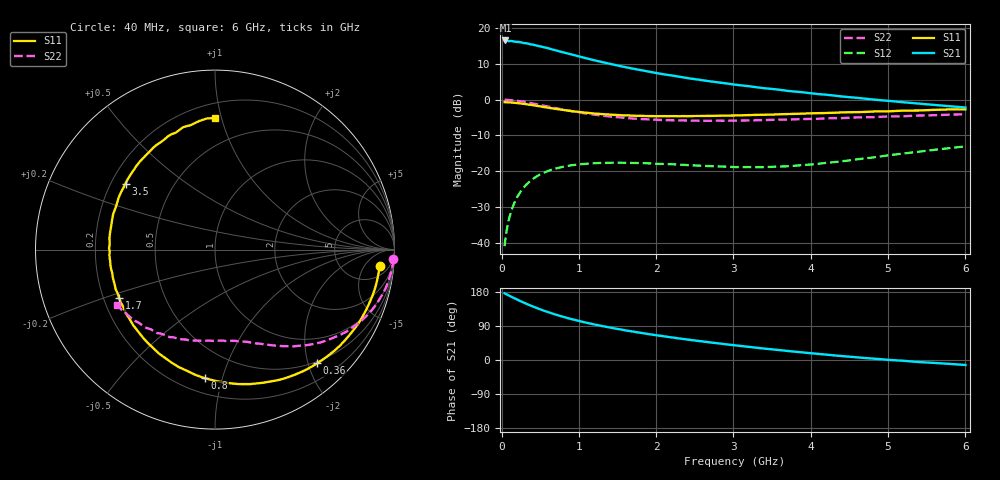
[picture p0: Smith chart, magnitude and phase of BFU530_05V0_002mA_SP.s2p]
! Filename:  P:\Prog\Test\Noise\ATS_data\Testdata_Net\03 Spar\BFU530_APG2013_40_A05_05p0V_002mA_SP_CM01_D.s2p
! Date/Time: Fri 26/Apr/2013 13:03:15
! BFU530_APG2013_40_A05_05p0V_1to25mA_SP_CM01_Bias2_R.s2p
! MDIF S-parameter v. bias file
! BFU530_APG2013_40_A05_05p0V_1to25mA_SP_CM01
! Date/time Wed Apr 24 19:36:53 2013
! VAR V_out= 5.0000
! VAR I_out= 1.9900
! VAR V_in= 0.7986
! VAR I_in= 0.0213
! Device data file deembeded for feedlines and parallel
! Original file: \03 Spar\BFU530_APG2013_40_A05_05p0V_002mA_SP_CM01_R.s2p
! Feed-files: PR047V01_250413_Feed1.s2p, PR047V01_250413_Feed2.s2p
! Parallel-file: PR047V01_250413_Par.s2p
# MHz S MA R 50
!  Freq-MHz  S11-mag  S11-arg  S21-mag  S21-arg  S12-mag  S12-arg  S22-mag  S22-arg
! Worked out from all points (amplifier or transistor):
!   98 points, 40 MHz to 6 GHz, reference 50 ohm
!   highest |S21| = 16.6 dB at 50 MHz (marker M1)
!   |S21| within 3 dB of that: start of sweep to 740.2 MHz
!   unconditionally stable (mu >= 1): 2.879 GHz to 4.826 GHz
!   at 300 MHz: K = 0.11, MSG = 20.0 dB, |S12| = -24.2 dB
!   at 1.6 GHz: K = 0.54, MSG = 13.4 dB, |S12| = -17.6 dB
!   at 6 GHz: K = 0.81, MSG = 5.4 dB, |S12| = -13.0 dB
!   S11 on the Smith chart (normalised r, x): 40 MHz: 10, -12; 360 MHz: 0.47, -2.16; 800 MHz: 0.30, -0.88; 1.7 GHz: 0.26, -0.22; 3.5 GHz: 0.26, +0.31; 6 GHz: 0.30, +0.95
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40  0.9241 -5.6  6.71 176.0  0.008973 86.3  0.9957 -3.0
50  0.9221 -6.9  6.73 174.4  0.01118 85.5  0.9959 -3.8
60  0.9208 -8.1  6.643 173.7  0.01341 84.9  0.9948 -4.7
120  0.9142 -16.6  6.629 167.6  0.02641 79.8  0.9843 -9.2
240  0.887 -32.8  6.374 155.8  0.05061 70.1  0.9517 -18.2
360  0.8517 -48.1  6.017 145.1  0.07123 61.4  0.9054 -26.2
440  0.8265 -57.6  5.761 138.4  0.08274 56.3  0.8706 -30.9
550  0.7886 -70.2  5.403 129.9  0.09555 49.7  0.8212 -36.8
700  0.7446 -85.4  4.905 119.8  0.109 42.3  0.7622 -43.5
800  0.7188 -94.6  4.589 113.8  0.1157 38.2  0.7258 -47.4
900  0.6928 -103.2  4.301 108.2  0.1211 34.5  0.6958 -50.8
1050  0.6642 -114.9  3.905 100.6  0.126 29.6  0.6518 -55.5
1200  0.6411 -125.4  3.562 93.8  0.1293 25.6  0.6183 -59.5
1350  0.6237 -134.6  3.265 87.7  0.131 22.4  0.5908 -63.1
1700  0.5981 -153.3  2.719 75.1  0.1305 17.0  0.5452 -70.5
2050  0.5887 -169.1  2.31 64.0  0.1268 13.9  0.5211 -77.4
2500  0.5918 173.9  1.939 51.5  0.1206 13.1  0.509 -85.8
3100  0.6043 154.3  1.585 36.9  0.1143 17.5  0.5118 -96.8
3500  0.6197 143.6  1.414 28.1  0.1155 22.7  0.5232 -104.2
4100  0.6483 128.0  1.198 16.0  0.1271 30.6  0.5413 -115.5
5200  0.705 104.5  0.921 -2.1  0.1772 35.9  0.5877 -135.9
6000  0.7332 90.2  0.7785 -13.1  0.2228 32.5  0.6262 -150.5
